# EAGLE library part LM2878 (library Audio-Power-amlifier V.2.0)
The LM2878 is a high voltage stereo power amplifier designed to deliver 5W/channel continuous into 8X loads. The amplifier is ideal for use with low regulation power supplies due to the absolute maximum rating of 35V and its superior power supply rejection.
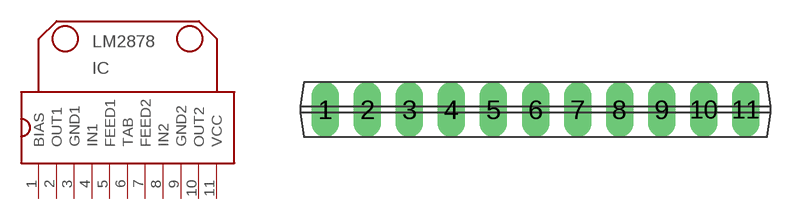
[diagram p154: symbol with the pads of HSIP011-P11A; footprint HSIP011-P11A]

Designator prefix IC

## LM2878  [HSIP011-P11A]
1  BIAS
2  OUT1  out
3  GND1  pwr
4  IN1  in
5  FEED1
6  TAB
7  FEED2
8  IN2  in
9  GND2  pwr
10  OUT2  out
11  VCC  pwr

## Footprint HSIP011-P11A (pad centres in mm)
Single-In-Line Package,NS Package Number P11A . http://www.ti.com/sc/docs/package/guide.htm
drill 1.1 long: 1 -12.7,0; 2 -10.16,0; 3 -7.62,0; 4 -5.08,0; 5 -2.54,0; 6 0,0; 7 2.54,0; 8 5.08,0; 9 7.62,0; 10 10.16,0; 11 12.7,0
